(* Logix 5000 AddOnInstructionDefinition export MSO_Yaskawa; software revision 17.00 *)

TYPE Yaskawa_EIP_Servo :   // Yaskawa SigmaLogic Axis Structure v2.4.0
STRUCT
   O : Yaskawa_OUT_to_Servo;
   I : Yaskawa_IN_from_Servo;
   AOI_SB : Yaskawa_AOI_Status_Bits;
END_STRUCT
END_TYPE

TYPE Yaskawa_OUT_to_Servo :   // Structure of data sent out to the Yaskawa SigmaLogic controller v2.4.0
STRUCT
   b00_ServoOn : BOOL;   // Servo On
   b01_Stop : BOOL;   // Stops All Current Motion in Progress
   b02_Home : BOOL;   // Start Homing Process
   b03_MoveStart1 : BOOL;   // Start Current Motion
   b06_SuperImpose : BOOL;
   b07_ServoAlarmReset : BOOL;   // Servo Alarm Reset
   b08_ControllerAlarmReset : BOOL;   // SigmaLogic Alarm Reset
   b09_MoveStart2 : BOOL;   // Start Second Motion (Blended Move)
   b10_MoveAbort : BOOL;   // Abort Current Move
   b11_MovePause : BOOL;   // Pause Current Move
   b12_SeqPause : BOOL;   // Indexing Sequence Pause
   b13_SeqResume : BOOL;   // Indexing Sequence Resume
   b14_SeqCancel : BOOL;   // Indexing Sequence Cancel
   b15_AbsEncoderReset : BOOL;   // Absolute Encoder Reset
   b16_SeqStart : BOOL;   // Start Indexing Sequence
   b17_SeqEditSpeed : BOOL;   // Enter Edit Speed
   b18_SeqEditDistance : BOOL;   // Enter Distance Edit
   b19_PLSEnable : BOOL;   // Enable PLS execution
   b20_PLSActivateOutput1 : BOOL;   // Activate PLS output1 switch logic
   b21_PLSActivateOutput2 : BOOL;   // Activate PLS output2 switch logic
   b22_PLSActivateOutput3 : BOOL;   // Activate PLS output3 switch logic
   b23_PLSActivateOutput4 : BOOL;   // Activate PLS output4 switch logic
   b24_SetClock : BOOL;   // Set the remote controller clock with data provided by the PLC
   RebootController : BOOL;
   UseExternalEncoder : BOOL;   // Use External Encoder when executing MAHSP_Yaskawa
   b32_HeatbeatAnswer : BOOL;   // Heartbeat Answer
   BrakeBypassRequest : BOOL;
   SetFwdTorqueLimit : BOOL;
   SetRevTorqueLimit : BOOL;
   TorqueLimit : DINT;
   TorqueRamp : DINT;
   HomeMethod : INT;
   HomeSpeed : DINT;
   HomeAccDec : DINT;   // Home Move Acceleration/Deceleration Rate
   HomeBackOffDistance : DINT;
   HomeCreepSpeed : DINT;
   HomeCreepDistanceLimit : DINT;
   HomeCreepTimeLimit : DINT;
   HomeOffsetDistance : DINT;
   HomeOffsetSpeed : DINT;
   HomePostion : DINT;
   HomeTorque : DINT;
   HomeInputNo : DINT;
   HomeApproachTimeLimit : DINT;
   HomeApproachDistLimit : DINT;
   HomeDirection : INT;
   HomeSwitchMode : INT;
   MoveType : INT;
   MoveDirection : INT;
   MoveAccel1 : DINT;
   MoveAccel2 : DINT;
   MoveDecel1 : DINT;
   MoveDecel2 : DINT;
   MoveSpeed1 : DINT;
   MoveSpeed2 : DINT;
   MoveDistance1 : DINT;
   MoveDistance2 : DINT;
   MovePosition1 : DINT;
   MovePosition2 : DINT;
   RegistrationDistance : DINT;
   GearNumerator : DINT;
   GearDenominator : DINT;
   SuperImposeDistance : DINT;
   Resolution : INT;
   RegistrationDirection : INT;
   TuningLevel : INT;
   SequenceStep : INT;   // Staring Sequence Step Number
   SequenceEditStep : INT;   // Sequence Step Number to Edit
   FlagCommandBits1 : DINT;   // Flag Commands. 1..64 are General Flags, Bits 0..31 correspond to Flag 1..32
   FlagCommandBits2 : DINT;   // Flag Commands cont. 1..64 are General Flags, Bits 0..31 correspond to Flag 33..64
   DigitalOutCommandBits : DINT;   // Digital Output commands. Bits 0-7 correspond to CN13 Digital Outputs 0-7, used as Flag 73-80. Bits 8-10 correspond to CN1 Digital Outputs 0-2 used as Flag 88-90"
   SequenceEditSpeed : DINT;
   SequenceEditDistance : DINT;
   FeedRateOverride : INT;
   HSI_Enable : BOOL;
   HSI_MoveMode : BOOL;   // 0=Relative; 1=Moves per Cycle
   HSI_CalcMethod : BOOL;   // 0=Accel/Decel; 1=Time
   HSI_MoveDirection : BOOL;   // 0 = Negative; 1 = Positive
   HSI_TriggerFlag : INT;
   HSI_MovingFlag : INT;
   HSI_DwellingFlag : INT;
   HSI_DoneFlag : INT;
   HSI_MoveType : INT;   // 0=Single; 1=Repeat; 2=Repeat "x" times
   HSI_RepeatNumber : INT;
   HSI_Distance : DINT;
   HSI_Speed : DINT;
   HSI_Accel : DINT;
   HSI_MoveTime : DINT;
   HSI_DwellTime : DINT;
   PLS_OutputFlag1 : INT;
   PLS_OutputFlag2 : INT;
   PLS_OutputFlag3 : INT;
   PLS_OutputFlag4 : INT;
   PLS_OnPosition1 : DINT;
   PLS_OffPosition1 : DINT;
   PLS_OnPosition2 : DINT;
   PLS_OffPosition2 : DINT;
   PLS_OnPosition3 : DINT;
   PLS_OffPosition3 : DINT;
   PLS_OnPosition4 : DINT;
   PLS_OffPosition4 : DINT;
   PLS_OnCompensation1 : INT;
   PLS_OffCompensation1 : INT;
   PLS_OnCompensation2 : INT;
   PLS_OffCompensation2 : INT;
   PLS_OnCompensation3 : INT;
   PLS_OffCompensation3 : INT;
   PLS_OnCompensation4 : INT;
   PLS_OffCompensation4 : INT;
   RTC_Year : INT;
   RTC_Month : INT;
   RTC_Day : INT;
   RTC_Hour : INT;
   RTC_Min : INT;
   RTC_Sec : INT;
   StopDecel : DINT;
   AnalogOutput : INT;   // CN13, AO_01 [mV]
END_STRUCT
END_TYPE

TYPE Yaskawa_AOI_Status_Bits :   // Internal bits used to interlock Yaskawa AOI execution. v2.4.0
STRUCT
   MAM : BOOL;   // Move AOI Active
   MAJ : BOOL;   // Jog AOI Active
   MAB : BOOL;   // Blending AOI Active
   MAG : BOOL;   // Gearing AOI Active
   MAHSP : BOOL;   // Home SetPoint AOI Active
   MAH : BOOL;   // Homing AOI Active
   MSQE : BOOL;   // Sequence Edit AOI Active
   MSQR : BOOL;   // Sequence Run AOI Active
   MHSI : BOOL;   // High Speed Index AOI Active
   MSO : BOOL;   // Servo On
   MSF : BOOL;   // Servo Off
   MAFR : BOOL;   // Fault Reset
   MAS : BOOL;   // Servo Abort
   MTRQ : BOOL;   // Torque Mode Active
   MPLS : BOOL;   // PLS Active
   MCLK : BOOL;   // SetClock Active
   MSTL : BOOL;   // Set Torque Limit Active
   AOI_Permissive : BOOL;   // Permissive to Execute an AOI
END_STRUCT
END_TYPE

TYPE Yaskawa_IN_from_Servo :   // Structure of data coming from the Yaskawa SigmaLogic controller. v2.4.0
STRUCT
   AlarmText : STRING;   // ServoPack Alarm Code plus Text Description
   b00_Heartbeat : BOOL;
   b01_Alarm : BOOL;   // ServoPack Alarm
   b02_Warning : BOOL;   // ServoPack Warning
   b03_Ready : BOOL;   // ServoPack Ready
   b04_Enabled : BOOL;   // ServoPack Enabled ("Servo On")
   b05_StopComplete : BOOL;
   b06_HomeComplete : BOOL;
   b07_HomeBusy : BOOL;
   b08_HomeActive : BOOL;
   b09_HomeAborted : BOOL;
   b10_HomeError : BOOL;
   b11_MoveAbsComplete : BOOL;
   b12_MoveAbsBusy : BOOL;
   b13_MoveAbsActive : BOOL;
   b14_MoveAbsAborted : BOOL;
   b15_MoveAbsError : BOOL;
   b16_MoveRelComplete : BOOL;
   b17_MoveRelBusy : BOOL;
   b18_MoveRelActive : BOOL;
   b19_MoveRelAborted : BOOL;
   b20_MoveRelError : BOOL;
   b21_JogAtSpeed : BOOL;
   b22_JogBusy : BOOL;
   b23_JogActive : BOOL;
   b24_JogAborted : BOOL;
   b25_JogError : BOOL;
   b26_GearInSync : BOOL;
   b27_GearBusy : BOOL;
   b28_GearActive : BOOL;
   b29_GearAborted : BOOL;
   b30_GearError : BOOL;
   b32_MoveSuperComplete : BOOL;
   b33_MoveSuperBusy : BOOL;
   b34_MoveSuperActive : BOOL;
   b35_MoveSuperAborted : BOOL;
   b36_MoveSuperError : BOOL;
   b37_PowerCycleRequired : BOOL;
   b38_MoveBlend1Complete : BOOL;
   b39_MoveBlend1Busy : BOOL;
   b40_MoveBlend1Active : BOOL;
   b41_MoveBlend1Abort : BOOL;
   b42_MoveBlend1Error : BOOL;
   b43_MoveBlend2Complete : BOOL;
   b44_MoveBlend2Busy : BOOL;
   b45_MoveBlend2Active : BOOL;
   b46_MoveBlend2Abort : BOOL;
   b47_MoveBlend2Error : BOOL;
   b48_RegComplete : BOOL;
   b49_RegBusy : BOOL;
   b50_RegActive : BOOL;
   b51_RegAborted : BOOL;
   b52_RegError : BOOL;
   b53_ResetAbsEncoderActive : BOOL;
   b54_ResetAbsEncoderBusy : BOOL;
   b55_ResetAbsEncoderDone : BOOL;
   b56_ResetAbsEncoderError : BOOL;
   b57_SeqRunning : BOOL;
   b58_RegSensorNotReached : BOOL;
   b59_SeqEditError : BOOL;
   b60_SeqEditDone : BOOL;
   b61_TorqueAtTorque : BOOL;
   b62_TorqueBusy : BOOL;
   b63_TorqueActive : BOOL;
   b64_TorqueAborted : BOOL;
   b65_TorqueError : BOOL;
   b66_ControllerAlarm : BOOL;
   b67_ApplicationError : BOOL;
   b68_AxisAtStandStill : BOOL;
   b69_TestModeActive : BOOL;
   b70_ServoParamsOK : BOOL;
   b71_SetFwdTorqueLimitDone : BOOL;
   b72_SetRevTorqueLimitDone : BOOL;
   Position : DINT;
   Speed : DINT;
   Torque : DINT;
   HomeErrorID : INT;
   MoveAbsErrorID : INT;
   MoveRelErrorID : INT;
   JogErrorID : INT;
   GearErrorID : INT;
   MoveSuperErrorID : INT;
   ServoAlarmID : INT;
   ServoWarningID : INT;
   ControllerAlarmID : DINT;
   AxisGenAlarmID : DINT;
   MoveBlend1ErrorID : INT;
   MoveBlend2ErrorID : INT;
   ResetAbsEncoderErrorID : INT;
   FunctionBlockErrorID : INT;
   TorqueErrorID : INT;
   RegErrorID : INT;
   SeqCurrentStep : INT;
   FlagStatusBit1 : DINT;   // Flag Status. 1..64 are General Flags, Bits 0..31 correspond to Flag 1..32
   FlagStatusBit2 : DINT;   // Flag Status cont. 1..64 are General Flags, Bits 0..31 correspond to Flag 33..64
   IOStatusBits : DINT;   // Digital IO Status. Bits 0-7, CN13 Inputs 0-7, Used as Flag 65-72. Bits 8-15, CN13 Outputs 0-7, Used as Flag 73-80. Bits 16-22, CN1 Inputs 0-6, Used as Flag 81-87. Bits 23-25, CN1 Outputs 0-4, Used as Flag 88-92.
   HSI_Moving : BOOL;
   HSI_Dwelling : BOOL;
   HSI_Done : BOOL;
   HSI_Busy : BOOL;
   HSI_Error : BOOL;
   HSI_ErrorCode : INT;
   PLS_Running : BOOL;
   PLS_SwitchStatus1 : BOOL;
   PLS_SwitchStatus2 : BOOL;
   PLS_SwitchStatus3 : BOOL;
   PLS_SwitchStatus4 : BOOL;
   PLS_Busy : BOOL;
   PLS_Error : BOOL;
   PLS_ErrorCode : INT;
   SetClock_Done : BOOL;
   SetClock_Busy : BOOL;
   SetClock_Error : BOOL;
   SetClock_ErrorID : INT;
   SoftwareVersion : DINT;
   FirmwareVersion : DINT;
   CommandedPos : DINT;
   CommandedPosNonCyc : DINT;
   CommandedSpeed : DINT;
   Clock_Year : INT;
   Clock_Month : INT;
   Clock_Day : INT;
   Clock_Hour : INT;
   Clock_Minute : INT;
   Clock_Second : INT;
   AnalogInput : REAL;   // CN13, AI_01 [v]
   BrakeBypassActive : BOOL;
   ForwardTorqueLimit : DINT;
   ReverseTorqueLimit : DINT;
END_STRUCT
END_TYPE

ADD_ON_INSTRUCTION MSO_Yaskawa   (* revision 2.4 0, vendor Yaskawa America, Inc., ExecuteEnableInFalse *)
// Motion Servo On
// Revision note:
// 2.4.0: No functional change
// 2.3.1: Moved unlatch of AOI_ON_LOCAL to bottom of EnableInFalse routine so that outputs will be on for at least 1 scan if one-shot on EN is used.
// 2.3.0: No functional change
// 2.0.0: No functional change.
// 1.2.0: No functional change.
// Initial Release 9/10/2014
// Help:
// The Motion Axis Servo On (MSO_Yaskawa) function activates the servo loop of a remote axis. This is also referred to as 'Enabling' the axis.
// The EN output will mirror the state of EnableIn (rung power)
// The DN output will come on after the command has been received and the servo axis is verified to be 'Enabled' and under servo loop control. This process may take several scans to complete.
// The FLT_RDY output will come on if conditions are not right for the axis to become enabled. Examples of this condition are:
// - Main power is not applied
// - The axis is faulted
// - Hardware BaseBlock (ST0) is applied
// The FLT_BSY output will be set ON if another Yaskawa AOI already has control. Control condition can be monitored at the MCFG_Yaskawa.AOI_Active output.
// Once the axis is enabled, the axis enabled status can be continuously monitored at MCFG_Yaskawa.SvON output.
// Releasing EnableIn will set all block outputs to OFF.
VAR_IN_OUT
   Axis : Yaskawa_EIP_Servo; {required}
END_VAR
VAR_OUTPUT
   EN : BOOL; {visible}   // Function is executing
   DN : BOOL; {visible}   // MSO completed successfully and the axis servo loop is Enabled
   FLT_RDY : BOOL; {visible}   // Conditions are not right for the function to properly complete.
   FLT_BSY : BOOL; {visible}   // Another Yaskawa AOI has control of the axis.
END_VAR
VAR
   AOI_ON_LOCAL : BOOL;
   Finished : BOOL;   // Function is Finished
END_VAR

ROUTINE EnableInFalse   (* ladder *)
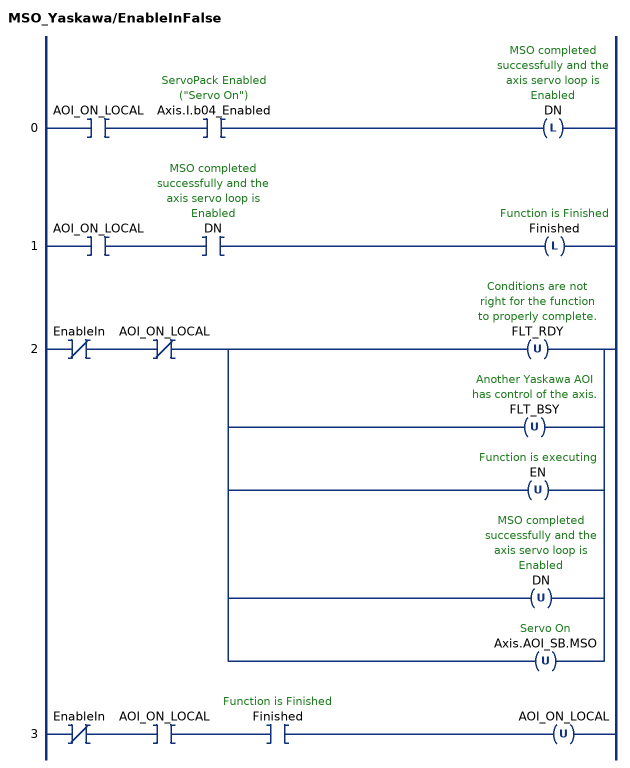
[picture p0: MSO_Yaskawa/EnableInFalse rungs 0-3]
   0: XIC(AOI_ON_LOCAL)XIC(Axis.I.b04_Enabled)OTL(DN);
   1: XIC(AOI_ON_LOCAL)XIC(DN)OTL(Finished);
   2: XIO(EnableIn)XIO(AOI_ON_LOCAL)[OTU(FLT_RDY) ,OTU(FLT_BSY) ,OTU(EN) ,OTU(DN) ,OTU(Axis.AOI_SB.MSO) ];
   3: XIO(EnableIn)XIC(AOI_ON_LOCAL)XIC(Finished)OTU(AOI_ON_LOCAL);
END_ROUTINE

ROUTINE Logic   (* ladder *)
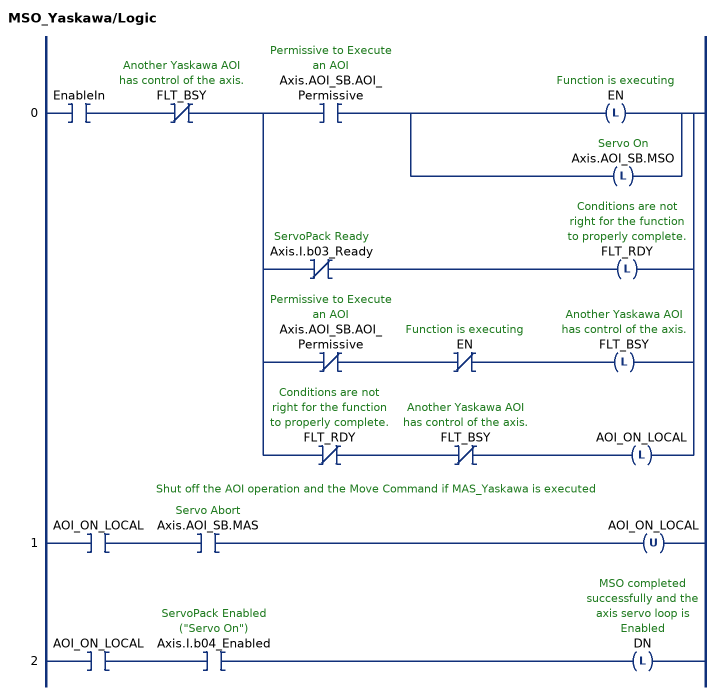
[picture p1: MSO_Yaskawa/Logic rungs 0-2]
   0: XIC(EnableIn)XIO(FLT_BSY)[XIC(Axis.AOI_SB.AOI_Permissive) [OTL(EN) ,OTL(Axis.AOI_SB.MSO) ] ,XIO(Axis.I.b03_Ready) OTL(FLT_RDY) ,XIO(Axis.AOI_SB.AOI_Permissive) XIO(EN) OTL(FLT_BSY) ,XIO(FLT_RDY) XIO(FLT_BSY) OTL(AOI_ON_LOCAL) ];
   // Shut off the AOI operation and the Move Command if MAS_Yaskawa is executed
   1: XIC(AOI_ON_LOCAL)XIC(Axis.AOI_SB.MAS)OTU(AOI_ON_LOCAL);
   2: XIC(AOI_ON_LOCAL)XIC(Axis.I.b04_Enabled)OTL(DN);
END_ROUTINE
END_ADD_ON_INSTRUCTION
